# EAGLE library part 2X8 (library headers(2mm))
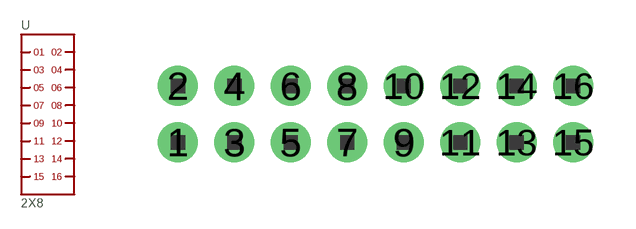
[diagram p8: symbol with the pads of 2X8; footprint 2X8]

Designator prefix -

## 2X8  [2X8]
1  1
2  2
3  3
4  4
5  5
6  6
7  7
8  8
9  9
10  10
11  11
12  12
13  13
14  14
15  15
16  16

## Footprint 2X8 (pad centres in mm)
drill 0.8 pad 1.422: 1 -7,-1; 2 -7,1; 3 -5,-1; 4 -5,1; 5 -3,-1; 6 -3,1; 7 -1,-1; 8 -1,1; 9 1,-1; 10 1,1; 11 3,-1; 12 3,1; 13 5,-1; 14 5,1; 15 7,-1; 16 7,1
